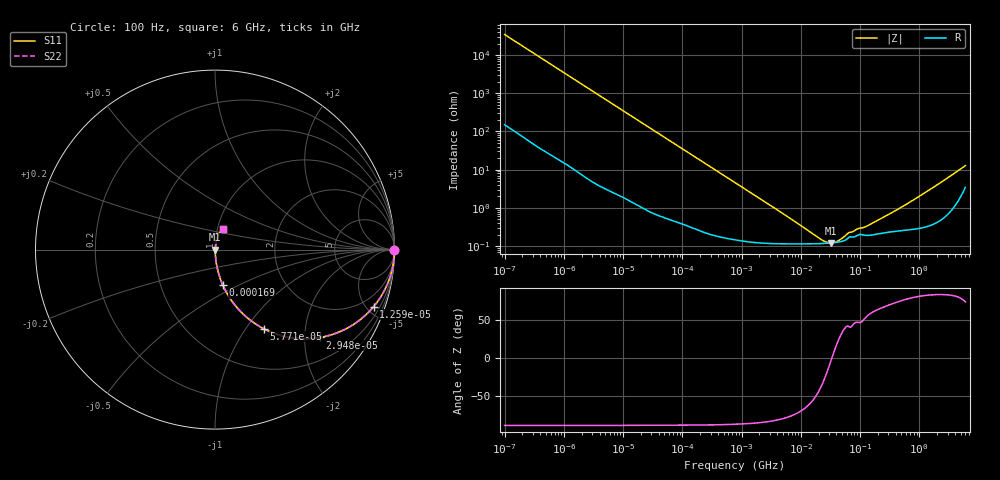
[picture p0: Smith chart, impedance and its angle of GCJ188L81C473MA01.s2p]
!Murata Part Number: GCJ188L81C473MA01
!These Parameters are Measured in Series Mode Connection
!Data Generated on Mar 13, 2026
!  o--ll--o
!Port1  Port2
!  o------o
!Operation Temp=25[degC], DC Bias Voltage=0[V]
!Freq. Start=100[Hz] Stop=6[GHz] 401[Steps]
# Hz S RI R 50
!Freq.(Hz) S11(Real) S11(Imag) S21(Real) S21(Imag) S12(Real) S12(Imag) S22(Real) S22(Imag)
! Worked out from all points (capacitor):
!   401 points, 100 Hz to 6 GHz, reference 50 ohm
!   read as one part in series: C = 46.1 nF near 109 Hz
!   lowest |Z| = 121 mohm at 31.85 MHz (marker M1)
!   series resonance near 33.47 MHz, so ESL is about 490 pH
!   S11 on the Smith chart (normalised r, x): 100 Hz: open; 12.59 kHz: 1.03, -5.55; 29.48 kHz: 1.02, -2.38; 57.71 kHz: 1.01, -1.22; 169 kHz: 1.01, -0.42; 6 GHz: 1.07, +0.25
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100  1 -0.0029  2.1e-05 0.0029  2.1e-05 0.0029  1 -0.0029
627  0.9996 -0.0181  0.000403 0.0181  0.000403 0.0181  0.9996 -0.0181
2008  0.9964 -0.0575  0.00357 0.0575  0.00357 0.0575  0.9964 -0.0575
5378  0.9761 -0.1505  0.0239 0.1505  0.0239 0.1505  0.9761 -0.1505
12592  0.8837 -0.3178  0.1163 0.3178  0.1163 0.3178  0.8837 -0.3178
18841  0.7739 -0.4154  0.2261 0.4154  0.2261 0.4154  0.7739 -0.4154
29482  0.5849 -0.4895  0.4151 0.4895  0.4151 0.4895  0.5849 -0.4895
40335  0.431 -0.4916  0.569 0.4916  0.569 0.4916  0.431 -0.4916
57709  0.2719 -0.4407  0.7281 0.4407  0.7281 0.4407  0.2719 -0.4407
94437  0.1246 -0.325  0.8754 0.325  0.8754 0.325  0.1246 -0.325
169018  0.0442 -0.1992  0.9558 0.1992  0.9558 0.1992  0.0442 -0.1992
330837  0.0132 -0.1055  0.9868 0.1055  0.9868 0.1055  0.0132 -0.1055
774597  0.00355 -0.0457  0.9964 0.0457  0.9964 0.0457  0.00355 -0.0457
1.555665e7  0.00115 -0.0018  0.9988 0.0018  0.9988 0.0018  0.00115 -0.0018
2.434276e7  0.00118 -0.000692  0.9988 0.000692  0.9988 0.000692  0.00118 -0.000692
3.184506e7  0.00121 -0.000107  0.9988 0.000107  0.9988 0.000107  0.00121 -0.000107
4.165952e7  0.00127 0.000476  0.9987 -0.000476  0.9987 -0.000476  0.00127 0.000476
6.518806e7  0.00171 0.0015  0.9983 -0.0015  0.9983 -0.0015  0.00171 0.0015
1.275994e8  0.00191 0.00267  0.9981 -0.00267  0.9981 -0.00267  0.00191 0.00267
3.124326e8  0.00237 0.0065  0.9976 -0.0065  0.9976 -0.0065  0.00237 0.0065
1.791126e9  0.00507 0.0354  0.9949 -0.0354  0.9949 -0.0354  0.00507 0.0354
6e9  0.047 0.1136  0.953 -0.1136  0.953 -0.1136  0.047 0.1136
